[IBIS ver]   3.2
[File name]   ads42xx.ibs
[File Rev]   2.0
[Date]   May 25, 2011
[Source]   Data created from TI-SPICE simulations
[Disclaimer] Property of Texas Instruments Incorporated.
   Unauthorized reproduction and/or distribution is strictly
   protected under copyright law. Created 2006, (C) Copyright
   2006, Texas Instruments Incorporated, All Rights Reserved
   UNLESS THERE IS A SIGNED, WRITTEN AGREEMENT TO THE CONTRARY,
   TEXAS INSTRUMENTS (TI) IS PROVIDING THE IBIS MODELS AND
   WITHOUT ANY WARRANTY, EXPRESSED OR IMPLIED. TI assumes no
   liability for: 1) the accuracy of the IBIS models provided to
   your company; 2) the proper functioning of these IBIS Models
   in your design or for any resulting applications; or 3)
   infringement of patents, copyrights or intellectual property
   rights resulting from your use of these IBIS models. TI
   provides IBIS Models as a service to our customers. You and
   your company shall not distribute, sell or give these models
   to anyone else without prior written permission from TI.
   TI reserves the right to make changes to our products or
   to discontinue any semiconductor product or service
   without notice, and advises our customers to obtain the
   latest version of relevant information to verify, before
   placing orders, that the information being relied on is
   current.
   Please be aware that your receipt and use of the IBIS
   information provided shall serve as acceptance of these
   terms and conditions.  If you do not accept these terms,
   you should return or destroy the IBIS models and any
   other accompanying information immediately.
[Notes]   Revision History:
   Rev 2.0: 05/25/2011
   - Added ads424x and ads422x components.
   - Original model released March 9, 2011
   This file contains IBIS Model of various buffers of
   ads42xx series of A/D converters generated with
   r_fixture of 50 ohm ( 100 ohm differential)
[Copyright]   Property of Texas Instruments Incorporated. Unauthorised
   reproduction and/or distribution is strictly prohibited. This
   product is protected under copyright law and trade secret law
   as an unpublished work. Created 2000,(C) Copyright 2000,Texas
   Instruments Inc., All Rights Reserved.These commodities are
   under the U.S. Government distribution license control.As
   such,they are not to be re-exported without the prior approval
   of the U.S. Department of Commerce.
|   Component ads424x
[Component] ads424x
[Manufacturer] Texas Instruments.
[Package]  |64-pin QFN package (RGC)
| variable   typ   min   max
R_pkg   0.60837   0.52897   0.78365
L_pkg   2.09208nH   1.78421nH   2.77432nH
C_pkg   0.17978pF   0.12083pF   0.27053pF
[Pin]   signal_name   model_name   R_pin   L_pin   C_pin
|   (ohms)   (nH)   (pF)
1   DRVDD   POWER   0.00665  0.18847n  1.55275p
2   DB4/DB4M   dataoutput   0.25978  3.46638n  0.26319p
3   DB5/DB4P   dataoutput   0.24064  3.19328n  0.26048p
4   DB6/DB6M   dataoutput   0.22712  3.00077n  0.24768p
5   DB7/DB6P   dataoutput   0.21271  2.79593n  0.23148p
6   DB8/DB8M   dataoutput   0.20376  2.66901n  0.22219p
7   DB9/DB8P   dataoutput   0.19623  2.56231n  0.21333p
8   DB10/DB10M   dataoutput   0.19351  2.52370n  0.21192p
9   DB11/DB10P   dataoutput   0.19443  2.53681n  0.21224p
10   DB12/DB12M   dataoutput   0.19851  2.59450n  0.21606p
11   DB13/DB12P   dataoutput   0.20766  2.72432n  0.22239p
|12   RESET   dummy   0.21101  2.77182n  0.21940p
|13   SCLK   dummy   0.22498  2.97037n  0.24168p
|14   SDATA   dummy   0.24192  3.21147n  0.26052p
|15   SEN   dummy   0.26121  3.48668n  0.27190p
16   AVDD   POWER   0.13160  2.69701n  0.34617p
17   AGND   GND   0.12590  2.76581n  0.30939p
18   AGND   GND   0.11043  2.34459n  0.28369p
|19   INP_B   dummy   0.11005  2.33369n  0.31002p
|20   INM_B   dummy   0.10386  2.16475n  0.31723p
21   AGND   GND   0.09874  2.02643n  0.30170p
22   AVDD   POWER   0.09491  1.92314n  0.28364p
|23   CM   dummy   0.18418  2.38690n  0.20626p
24   AGND   GND   0.09181  1.83786n  0.25661p
25   CLKP   input   0.09190  1.84028n  0.26249p
26   CLKM   input   0.09340  1.87848n  0.26215p
27   AGND   GND   0.18678  2.42191n  0.19913p
28   AGND   GND   0.09738  1.98241n  0.28929p
|29   INP_A   dummy   0.10211  2.10766n  0.31190p
|30   INM_A   dummy   0.10798  2.26515n  0.32175p
31   AGND   GND   0.23068  3.04398n  0.26026p
32   AGND   GND   0.12379  2.73611n  0.31925p
33   AGND   GND   0.11731  2.28627n  0.31332p
34   AGND   GND   0.22454  2.95568n  0.22775p
|35   CTRL1   dummy   0.21569  2.82919n  0.22392p
|36   CTRL2   dummy   0.20163  2.62887n  0.21656p
|37   CTRL3   dummy   0.19139  2.48333n  0.19614p
|38   NC   dummy   0.20133  2.62451n  0.21209p
|39   NC   dummy   0.19120  2.48051n  0.20530p
40   DB13/DB12P   dataoutput   0.18595  2.40600n  0.20034p
41   DB13/DB12P   dataoutput   0.18494  2.39171n  0.20346p
42   DB13/DB12P   dataoutput   0.18751  2.42820n  0.20401p
43   DB13/DB12P   dataoutput   0.19515  2.53672n  0.21437p
44   DB13/DB12P   dataoutput   0.20431  2.66692n  0.22403p
45   DB13/DB12P   dataoutput   0.21909  2.87737n  0.24069p
46   DB13/DB12P   dataoutput   0.23294  3.07499n  0.25401p
47   DB13/DB12P   dataoutput   0.25251  3.35458n  0.25831p
48   DRVDD   POWER   0.12014  2.62871n  0.29108p
49   DRGND   GND   0.12334  2.73192n  0.30136p
50   DA8/DB8M   dataoutput   0.23167  3.05778n  0.25324p
51   DA9/DB8P   dataoutput   0.21378  2.80328n  0.23217p
52   DA10/DB10M   dataoutput   0.20166  2.63157n  0.22602p
53   DA11/DB10P   dataoutput   0.18968  2.46233n  0.21229p
54   DA12/DB12M   dataoutput   0.18326  2.37221n  0.20125p
55   DA13/DB12P   dataoutput   0.17966  2.32201n  0.19871p
56   NC/CLKOUTM   clockoutm   0.18046  2.33410n  0.19832p
57   CLKOUT/CLKOUP clockoutp   0.18598  2.41331n  0.19577p
|58   NC   dummy   0.18114  2.34400n  0.19616p
|59   NC   dummy   0.18763  2.43682n  0.20338p
60   DB0/DB0M   dataoutput   0.19781  2.58192n  0.21503p
61   DB1/DB0P   dataoutput   0.21244  2.79047n  0.23458p
62   DB2/DB2P   dataoutput   0.22626  2.98769n  0.24830p
63   DB3/DB2P   dataoutput   0.24585  3.26768n  0.25702p
64   SDOUT   dataoutput   0.25429  3.39084n  0.23272p
[Diff Pin]   inv_pin   vdiff   tdelay_typ   tdelay_min   tdelay_max
  3   2   350mV   0   0   0
  5   4   350mV   0   0   0
  7   6   350mV   0   0   0
  9   8   350mV   0   0   0
  11   10   350mV   0   0   0
  41   40   350mV   0   0   0
  43   42   350mV   0   0   0
  45   44   350mV   0   0   0
  47   46   350mV   0   0   0
  51   50   350mV   0   0   0
  53   52   350mV   0   0   0
  55   54   350mV   0   0   0
  61   60   350mV   0   0   0
  63   62   350mV   0   0   0
  57   56   350mV   0   0   0
  25   26   350mV   0   0   0
|   Component ads422x
[Component] ads422x
[Manufacturer] Texas Instruments.
[Package]   |64-pin QFN package (RGC)
| variable   typ   min   max
R_pkg   0.60837   0.52897   0.78365
L_pkg   2.09208nH   1.78421nH   2.77432nH
C_pkg   0.17978pF   0.12083pF   0.27053pF
[Pin]   signal_name   model_name   R_pin   L_pin   C_pin
|   (ohms)   (nH)   (pF)
1   DRVDD   POWER   0.00665  0.18847n  1.55275p
2   DB2/DB2M   dataoutput   0.25978  3.46638n  0.26319p
3   DB3/DB2P   dataoutput   0.24064  3.19328n  0.26048p
4   DB4/DB4M   dataoutput   0.22712  3.00077n  0.24768p
5   DB5/DB4P   dataoutput   0.21271  2.79593n  0.23148p
6   DB6/DB6M   dataoutput   0.20376  2.66901n  0.22219p
7   DB7/DB6P   dataoutput   0.19623  2.56231n  0.21333p
8   DB8/DB8M   dataoutput   0.19351  2.52370n  0.21192p
9   DB9/DB8P   dataoutput   0.19443  2.53681n  0.21224p
10   DB10/DB10M   dataoutput   0.19851  2.59450n  0.21606p
11   DB11/DB10P   dataoutput   0.20766  2.72432n  0.22239p
16   AVDD   POWER   0.13160  2.69701n  0.34617p
17   AGND   GND   0.12590  2.76581n  0.30939p
18   AGND   GND   0.11043  2.34459n  0.28369p
|19   INP_B   dummy   0.11005  2.33369n  0.31002p
|20   INM_B   dummy   0.10386  2.16475n  0.31723p
21   AGND   GND   0.09874  2.02643n  0.30170p
22   AVDD   POWER   0.09491  1.92314n  0.28364p
|23   CM   dummy   0.18418  2.38690n  0.20626p
24   AGND   GND   0.09181  1.83786n  0.25661p
25   CLKP   input   0.09190  1.84028n  0.26249p
26   CLKM   input   0.09340  1.87848n  0.26215p
27   AGND   GND   0.18678  2.42191n  0.19913p
28   AGND   GND   0.09738  1.98241n  0.28929p
|29   INP_A   dummy   0.10211  2.10766n  0.31190p
|30   INM_A   dummy   0.10798  2.26515n  0.32175p
31   AGND   GND   0.23068  3.04398n  0.26026p
32   AGND   GND   0.12379  2.73611n  0.31925p
33   AGND   GND   0.11731  2.28627n  0.31332p
34   AGND   GND   0.22454  2.95568n  0.22775p
|35   CTRL1   dummy   0.21569  2.82919n  0.22392p
|36   CTRL2   dummy   0.20163  2.62887n  0.21656p
|37   CTRL3   dummy   0.19139  2.48333n  0.19614p
|38   NC   dummy   0.20133  2.62451n  0.21209p
|39   NC   dummy   0.19120  2.48051n  0.20530p
|40   NC   dummy   0.18595  2.40600n  0.20034p
|41   NC   dummy   0.18494  2.39171n  0.20346p
42   DB13/DB12P   dataoutput   0.18751  2.42820n  0.20401p
43   DB13/DB12P   dataoutput   0.19515  2.53672n  0.21437p
44   DB13/DB12P   dataoutput   0.20431  2.66692n  0.22403p
45   DB13/DB12P   dataoutput   0.21909  2.87737n  0.24069p
46   DB13/DB12P   dataoutput   0.23294  3.07499n  0.25401p
47   DB13/DB12P   dataoutput   0.25251  3.35458n  0.25831p
48   DRVDD   POWER   0.12014  2.62871n  0.29108p
49   DRGND   GND   0.12334  2.73192n  0.30136p
50   DA8/DB8M   dataoutput   0.23167  3.05778n  0.25324p
51   DA9/DB8P   dataoutput   0.21378  2.80328n  0.23217p
52   DA10/DB10M   dataoutput   0.20166  2.63157n  0.22602p
53   DA11/DB10P   dataoutput   0.18968  2.46233n  0.21229p
54   DA12/DB12M   dataoutput   0.18326  2.37221n  0.20125p
55   DA13/DB12P   dataoutput   0.17966  2.32201n  0.19871p
56   NC/CLKOUTM   clockoutm   0.18046  2.33410n  0.19832p
57   CLKOUT/CLKOUP clockoutp   0.18598  2.41331n  0.19577p
|58   NC   dummy   0.18114  2.34400n  0.19616p
|59   NC   dummy   0.18763  2.43682n  0.20338p
|60   NC   dummy   0.19781  2.58192n  0.21503p
|61   NC   dummy   0.21244  2.79047n  0.23458p
62   DB0/DB0M   dataoutput   0.22626  2.98769n  0.24830p
63   DB1/DB0P   dataoutput   0.24585  3.26768n  0.25702p
64   SDOUT   dataoutput   0.25429  3.39084n  0.23272p
[Diff Pin]   inv_pin   vdiff   tdelay_typ   tdelay_min   tdelay_max
  3   2   350mV   0   0   0
  5   4   350mV   0   0   0
  7   6   350mV   0   0   0
  9   8   350mV   0   0   0
  11   10   350mV   0   0   0
  43   42   350mV   0   0   0
  45   44   350mV   0   0   0
  47   46   350mV   0   0   0
  51   50   350mV   0   0   0
  53   52   350mV   0   0   0
  55   54   350mV   0   0   0
  63   62   350mV   0   0   0
  57   56   350mV   0   0   0
  25   26   350mV   0   0   0
[Series Pin Mapping]  pin_2   model_name
  25   26   series_cap
[Model Selector] clockoutp
|The clock output can be in lvds mode or cmos mode. In lvds mode the
|clock signal ia a differential signal between pins CLKOUTP and CLKOUTM
|and in cmos mode its a single ended signal at pin CLKOUTP only.
|Note that the model for cmos buffer is different for data and clock output
|buffers whereas the model for the lvds buffer is the same
|  Model name   Description
LVDS   LVDS 3-state buffer.
LVDS2X   LVDS 3-state buffer with 2X strength.
cmos_clk_low   CMOS 3-state (low strength) buffer.
cmos_clk_low1   CMOS 3-state (low1 strength) buffer.
cmos_clk_high   CMOS 3-state (high strength) buffer.
cmos_clk_high1  CMOS 3-state (high1 strength) buffer.
[Model Selector] clockoutm
|When the clock is output in the cmos mode, CLOCKOUTM is SCAN or
|register read. In the lvds mode the clock output is a differential
|signal between pins CLKOUTP and CLKOUTM.
|  Model name   Description
LVDS   LVDS 3-state buffer.
LVDS2X   LVDS 3-state buffer with 2X strength.
[Model Selector] dataoutput
|Note that the model for cmos buffer is different for data and clock output
|buffers whereas lvds buffer is the same
|  Model name
LVDS   LVDS 3-state buffer.
LVDS2X   LVDS 3-state buffer.
cmos_data_high1  CMOS 3-state (high1 strength) buffer.
|   Model series_cap
[Model]   series_cap
Model_type   Series
C_comp   2.00pF   2.00pF   2.00pF
[Temperature Range]   27.00   125.00   -40.00
[Voltage Range]   3.30V   3.00V   3.60V
[C Series]   6.42pF   5.44pF   7.4pF
| End [Model] series_cap
|End [Component]
| Models and submodels in the file (9): LVDS (3-state), LVDS2X (3-state), cmos_clk_low (3-state), cmos_clk_low1 (3-state), cmos_clk_high (3-state), cmos_clk_high1 (3-state), cmos_data_high1 (3-state), input (Terminator), series_cap (Series)
